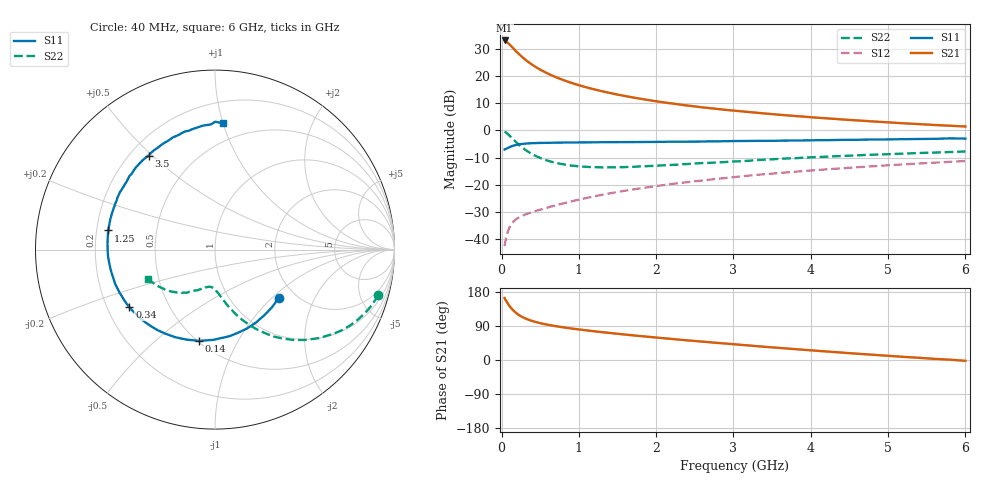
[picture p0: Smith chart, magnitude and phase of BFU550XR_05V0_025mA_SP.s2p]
! Filename:  P:\Prog\Test\Noise\ATS_data\Testdata_Net\03 Spar\BFU550XR_APG2013_45_C05_05p0V_025mA_SP_CM01_D.s2p
! Date/Time: Tue 06/Aug/2013 14:38:16
! BFU550XR_APG2013_45_C05_05p0V_25to35mA_SP_CM01_Bias1_R.s2p
! MDIF S-parameter v. bias file
! BFU550XR_APG2013_45_C05_05p0V_25to35mA_SP_CM01
! Date/time Mon Aug 05 16:56:59 2013
! bias mode 1
! bias variable = I_out
! VAR bias_var= 1
! VAR V_out= 5.0000
! VAR I_out= 25.0000
! VAR V_in= 0.8325
! VAR I_in= 0.2793
! Device data file deembeded for feedlines and parallel
! Original file: \03 Spar\BFU550XR_APG2013_45_C05_05p0V_025mA_SP_CM01_R.s2p
! Feed-files: PR006V01_02082013_Feed1.s2p, PR006V01_02082013_Feed2.s2p
! Parallel-file: PR006V01_02082013_Par.s2p
# MHz S MA R 50
!  Freq-MHz  S11-mag  S11-arg  S21-mag  S21-arg  S12-mag  S12-arg  S22-mag  S22-arg
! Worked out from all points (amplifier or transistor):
!   98 points, 40 MHz to 6 GHz, reference 50 ohm
!   highest |S21| = 33.0 dB at 40 MHz (marker M1)
!   |S21| within 3 dB of that: start of sweep to 155.2 MHz
!   unconditionally stable (mu >= 1): 1.333 GHz to 3.11 GHz
!   at 300 MHz: K = 0.51, MSG = 28.6 dB, |S12| = -31.0 dB
!   at 1.6 GHz: K = 1.02, MAG = 16.5 dB, |S12| = -22.2 dB
!   at 6 GHz: K = 0.86, MSG = 6.3 dB, |S12| = -11.3 dB
!   S11 on the Smith chart (normalised r, x): 40 MHz: 1.65, -1.10; 140 MHz: 0.51, -0.70; 340 MHz: 0.29, -0.28; 1.25 GHz: 0.25, +0.08; 3.5 GHz: 0.27, +0.49; 6 GHz: 0.36, +1.00
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40  0.4457 -36.9  44.84 163.5  0.007443 77.0  0.9443 -15.7
50  0.4517 -45.2  43.74 159.2  0.009128 75.2  0.9275 -19.5
80  0.4741 -67.8  40.68 149.5  0.0136 67.8  0.8611 -29.6
90  0.4804 -74.2  39.41 146.3  0.01488 65.7  0.835 -32.7
120  0.5029 -91.0  35.86 138.1  0.0181 60.5  0.7585 -40.6
140  0.5161 -99.9  33.51 133.4  0.01985 57.8  0.7101 -45.2
180  0.5361 -114.5  29.19 125.6  0.02269 53.8  0.6239 -52.6
220  0.551 -125.4  25.69 119.4  0.02481 51.5  0.5527 -58.3
280  0.5655 -137.4  21.49 112.3  0.02734 49.8  0.4699 -64.8
340  0.5747 -146.0  18.35 107.0  0.02954 49.5  0.4097 -69.6
400  0.5799 -152.8  15.96 102.7  0.03143 49.9  0.3629 -73.4
460  0.5849 -157.8  14.08 99.4  0.03357 50.6  0.3296 -76.3
650  0.5922 -169.8  10.22 91.1  0.04005 53.6  0.2641 -83.0
850  0.5978 -178.1  7.918 84.7  0.0474 56.2  0.2307 -88.2
1050  0.6003 175.3  6.445 79.4  0.05527 58.1  0.2154 -91.8
1250  0.6039 169.8  5.438 74.7  0.06332 59.2  0.2102 -95.6
2050  0.6158 152.0  3.339 58.4  0.0965 59.2  0.2263 -107.2
3100  0.637 132.2  2.238 40.0  0.1427 54.9  0.2712 -120.4
3500  0.6416 125.2  1.985 33.3  0.1603 52.0  0.2936 -125.4
4100  0.6584 115.1  1.701 24.0  0.1872 48.0  0.3234 -132.7
5200  0.6883 97.8  1.347 8.3  0.2368 39.4  0.3736 -146.3
6000  0.7057 86.5  1.177 -2.1  0.2728 32.3  0.4088 -156.5
